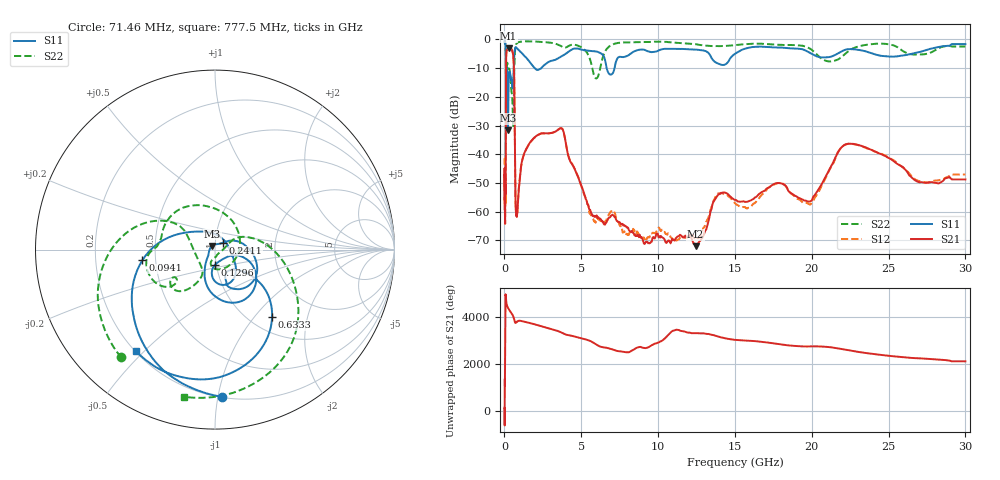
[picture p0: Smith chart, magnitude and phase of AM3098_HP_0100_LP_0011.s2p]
! Date/Time: Thu, Feb 28, 2019 8:35 AM
! Network Analyzer: Agilent Technologies E8364B Rev: A.07.50.67
! Sweep from 0.010 to 30.000 GHz, 1601 Points, Sweep Type: LOG
! Power Supply: 5.022 V, 0.002 A
# Hz S DB R 50
!freq MagS11 AngS11 MagS21 AngS21 MagS12 AngS12 MagS22 AngS22
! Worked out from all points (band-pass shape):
!   1601 points, 10 MHz to 30 GHz, reference 50 ohm
!   highest |S21| = -3.05 dB at 269.1 MHz (marker M1); lowest = -72.0 dB at 12.43 GHz (marker M2)
!   |S21| within 3 dB of the highest: 111.2 MHz to 576.6 MHz (465.4 MHz wide, 135 % of centre)
!   lowest |S11| = -31.7 dB at 229.3 MHz (marker M3), VSWR 1.05, Z = 48.4 + j1.99 ohm
!   |S11| at or under -10 dB: 175.9 MHz to 598.4 MHz (422.5 MHz wide, 109 % of centre); 1.975 GHz to 2.396 GHz (420.8 MHz wide, 19.3 % of centre); 6.651 GHz to 7.163 GHz (512.2 MHz wide, 7.41 % of centre)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
!   |S22| runs from -30.7 to -0.5 dB; largest |S21 - S12| = 0.0097
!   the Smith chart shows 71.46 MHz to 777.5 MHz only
!   S11 on the Smith chart (normalised r, x): 71.46 MHz: 0.20, -1.03; 94.1 MHz: 0.42, -0.06; 129.6 MHz: 0.98, -0.17; 241.1 MHz: 1.09, +0.09; 633.3 MHz: 1.25, -1.24; 777.5 MHz: 0.20, -0.47
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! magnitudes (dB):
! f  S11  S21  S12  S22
! 10 MHz  -0.3  -47.2  -41.3  -0.5
! 38.04 MHz  -0.5  -61.7  -59.8  -0.8
! 71.46 MHz  -1.7  -52.5  -52.5  -2.0
! 94.1 MHz  -7.8  -20.9  -20.8  -9.3
! 129.6 MHz  -21.2  -4.3  -4.3  -10.9
! 144.7 MHz  -15.6  -3.7  -3.7  -10.8
! 186.8 MHz  -11.2  -3.5  -3.5  -8.2
! 229.3 MHz  -31.7  -3.1  -3.1  -9.8
! 241.1 MHz  -24.5  -3.1  -3.1  -10.0
! 269.1 MHz  -14.8  -3.0  -3.0  -10.3
! 550.5 MHz  -15.9  -5.0  -4.9  -27.1
! 633.3 MHz  -6.2  -13.6  -13.5  -12.1
! 717.7 MHz  -2.7  -55.0  -56.1  -2.4
! 777.5 MHz  -2.9  -61.1  -61.0  -1.5
! 2.084 GHz  -10.5  -33.6  -33.7  -0.7
! 3.723 GHz  -5.9  -31.0  -31.0  -2.4
! 7.926 GHz  -5.9  -65.2  -67.9  -1.0
! 12.43 GHz  -3.5  -72.0  -69.2  -1.6
! 14.09 GHz  -8.8  -53.4  -53.7  -2.3
! 19.8 GHz  -4.4  -56.5  -57.4  -3.0
! 22.56 GHz  -3.4  -36.4  -36.4  -3.5
! 30 GHz  -1.6  -48.8  -47.1  -2.4
